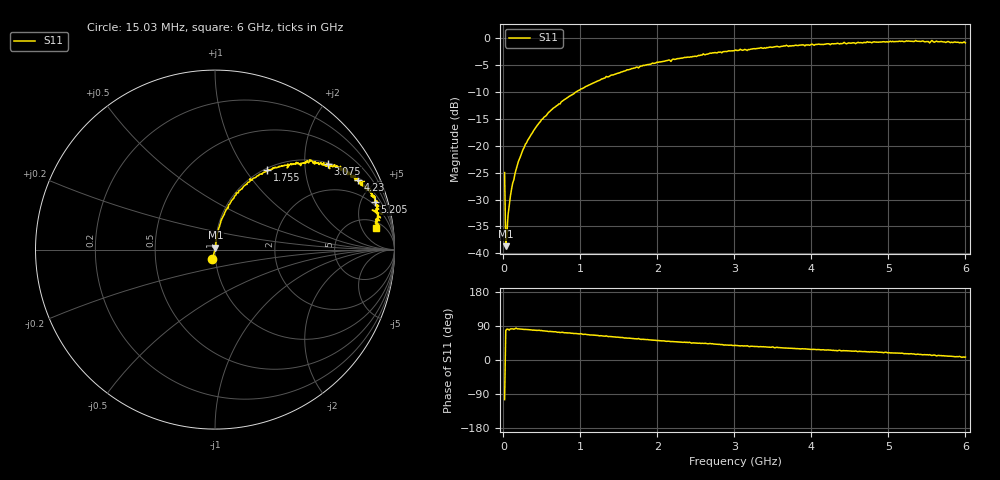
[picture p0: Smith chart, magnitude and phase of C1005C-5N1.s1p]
!	Network	Analyzer	HP8753E.07.74:	Oct	30	2002	Serial	No.	JP38451487
!	Hewlett-Packard
!	7	Sep	2009	8:28:23
!	Frequency	S11
#	HZ	S	RI	R	50
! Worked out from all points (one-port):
!   400 points, 15.03 MHz to 6 GHz, reference 50 ohm
!   lowest |S11| = -38.7 dB at 30.03 MHz (marker M1), VSWR 1.02, Z = 50.2 + j1.15 ohm
!   |S11| at or under -10 dB: start of sweep to 942 MHz
!   S11 on the Smith chart (normalised r, x): 15.03 MHz: 0.97, -0.11; 1.755 GHz: 1.03, +1.26; 3.075 GHz: 1.04, +2.61; 4.23 GHz: 1.11, +4.02; 5.205 GHz: 1.71, +6.44; 6 GHz: 7, +10
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1.502992e7  -0.0142 -0.0545
3.002985e7  0.00243 0.0114
6.00297e7  0.0035 0.0225
1.050295e8  0.00539 0.0391
1.95029e8  0.00975 0.0711
2.400288e8  0.0133 0.0858
4.950275e8  0.0368 0.171
7.650262e8  0.0754 0.249
1.065025e9  0.133 0.328
1.515022e9  0.243 0.412
1.755021e9  0.29 0.442
2.265019e9  0.434 0.479
3.015015e9  0.607 0.484
3.075015e9  0.629 0.476
3.165014e9  0.608 0.47
3.765011e9  0.729 0.435
4.230009e9  0.795 0.39
4.515007e9  0.821 0.361
4.935005e9  0.877 0.303
4.965005e9  0.861 0.326
5.205004e9  0.889 0.264
5.265004e9  0.904 0.264
5.445003e9  0.916 0.224
5.535002e9  0.876 0.22
5.565002e9  0.931 0.199
5.595002e9  0.892 0.21
5.625002e9  0.922 0.177
6e9  0.896 0.12
